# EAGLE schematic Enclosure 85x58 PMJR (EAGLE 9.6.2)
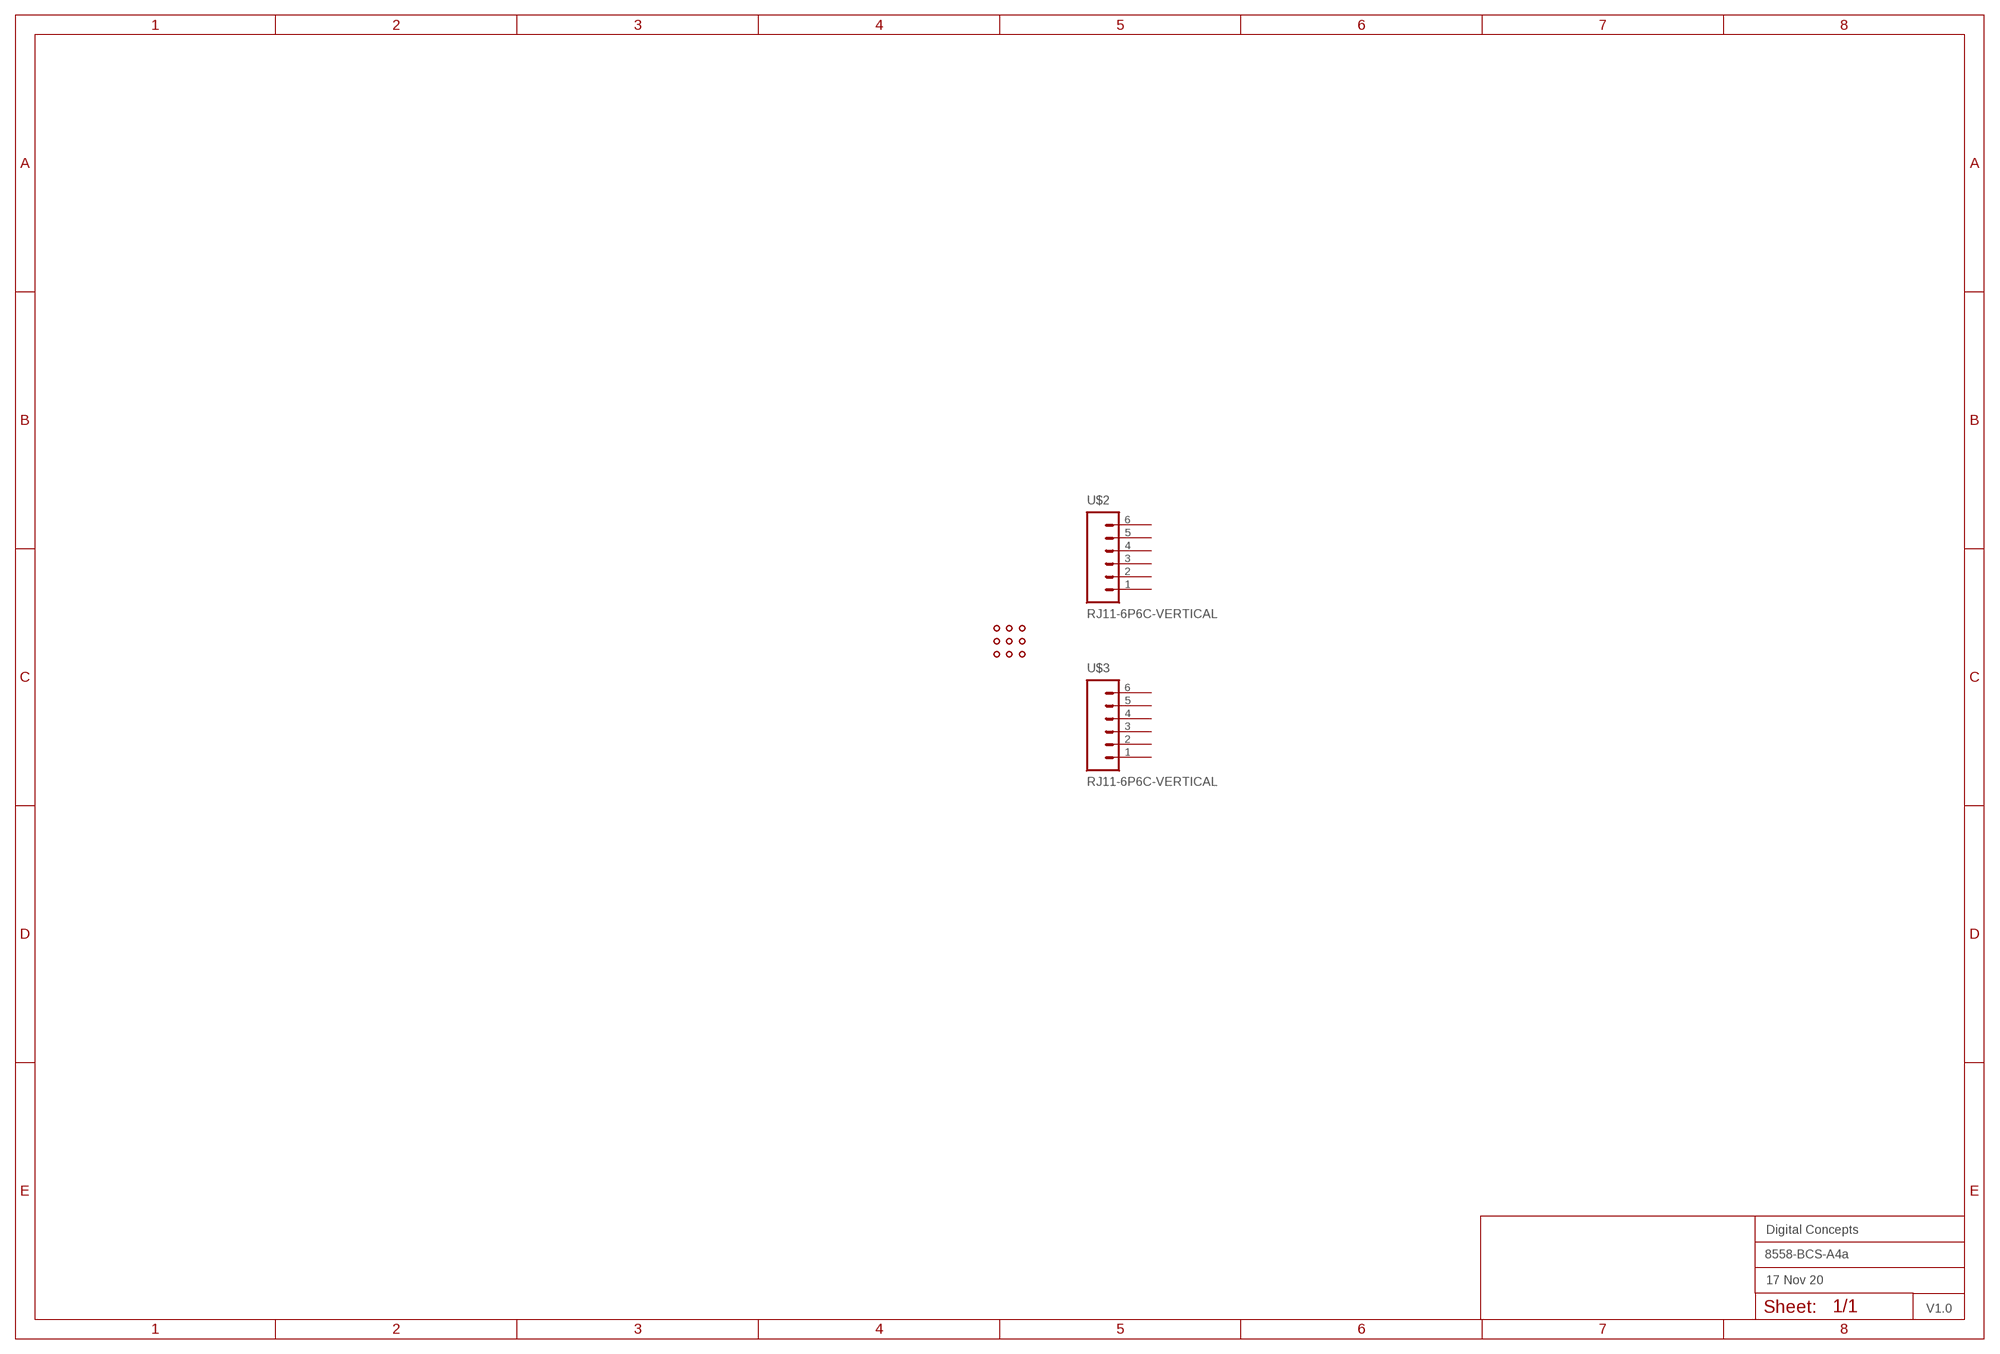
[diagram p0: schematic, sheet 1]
FRAME2 (A3L-LOC): DATE: 17 Nov 20; OWNER: Digital Concepts; TITLE: 8558-BCS-A4a; VERSION: V1.0

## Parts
U$1  PROTO-28X18-JST-RJ  [PROTO-28X18-JST-RJ]
U$2  RJ11-6P6C-VERTICAL  [RJ11-6-VERTICAL]
U$3  RJ11-6P6C-VERTICAL  [RJ11-6-VERTICAL]
Unconnected: U$2.1 U$2.2 U$2.3 U$2.4 U$2.5 U$2.6 U$3.1 U$3.2 U$3.3 U$3.4 U$3.5 U$3.6

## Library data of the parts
U$1 = digitalconcepts:PROTO-28X18-JST-RJ: 28 x 18 Prototyping board with JST pads and space for RJ11 sockets to fit an 85 x 58 enclosure
U$2 U$3 = digitalconcepts:RJ11-6P6C-VERTICAL: RJ11-6P6C-Vertical PCB Socket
